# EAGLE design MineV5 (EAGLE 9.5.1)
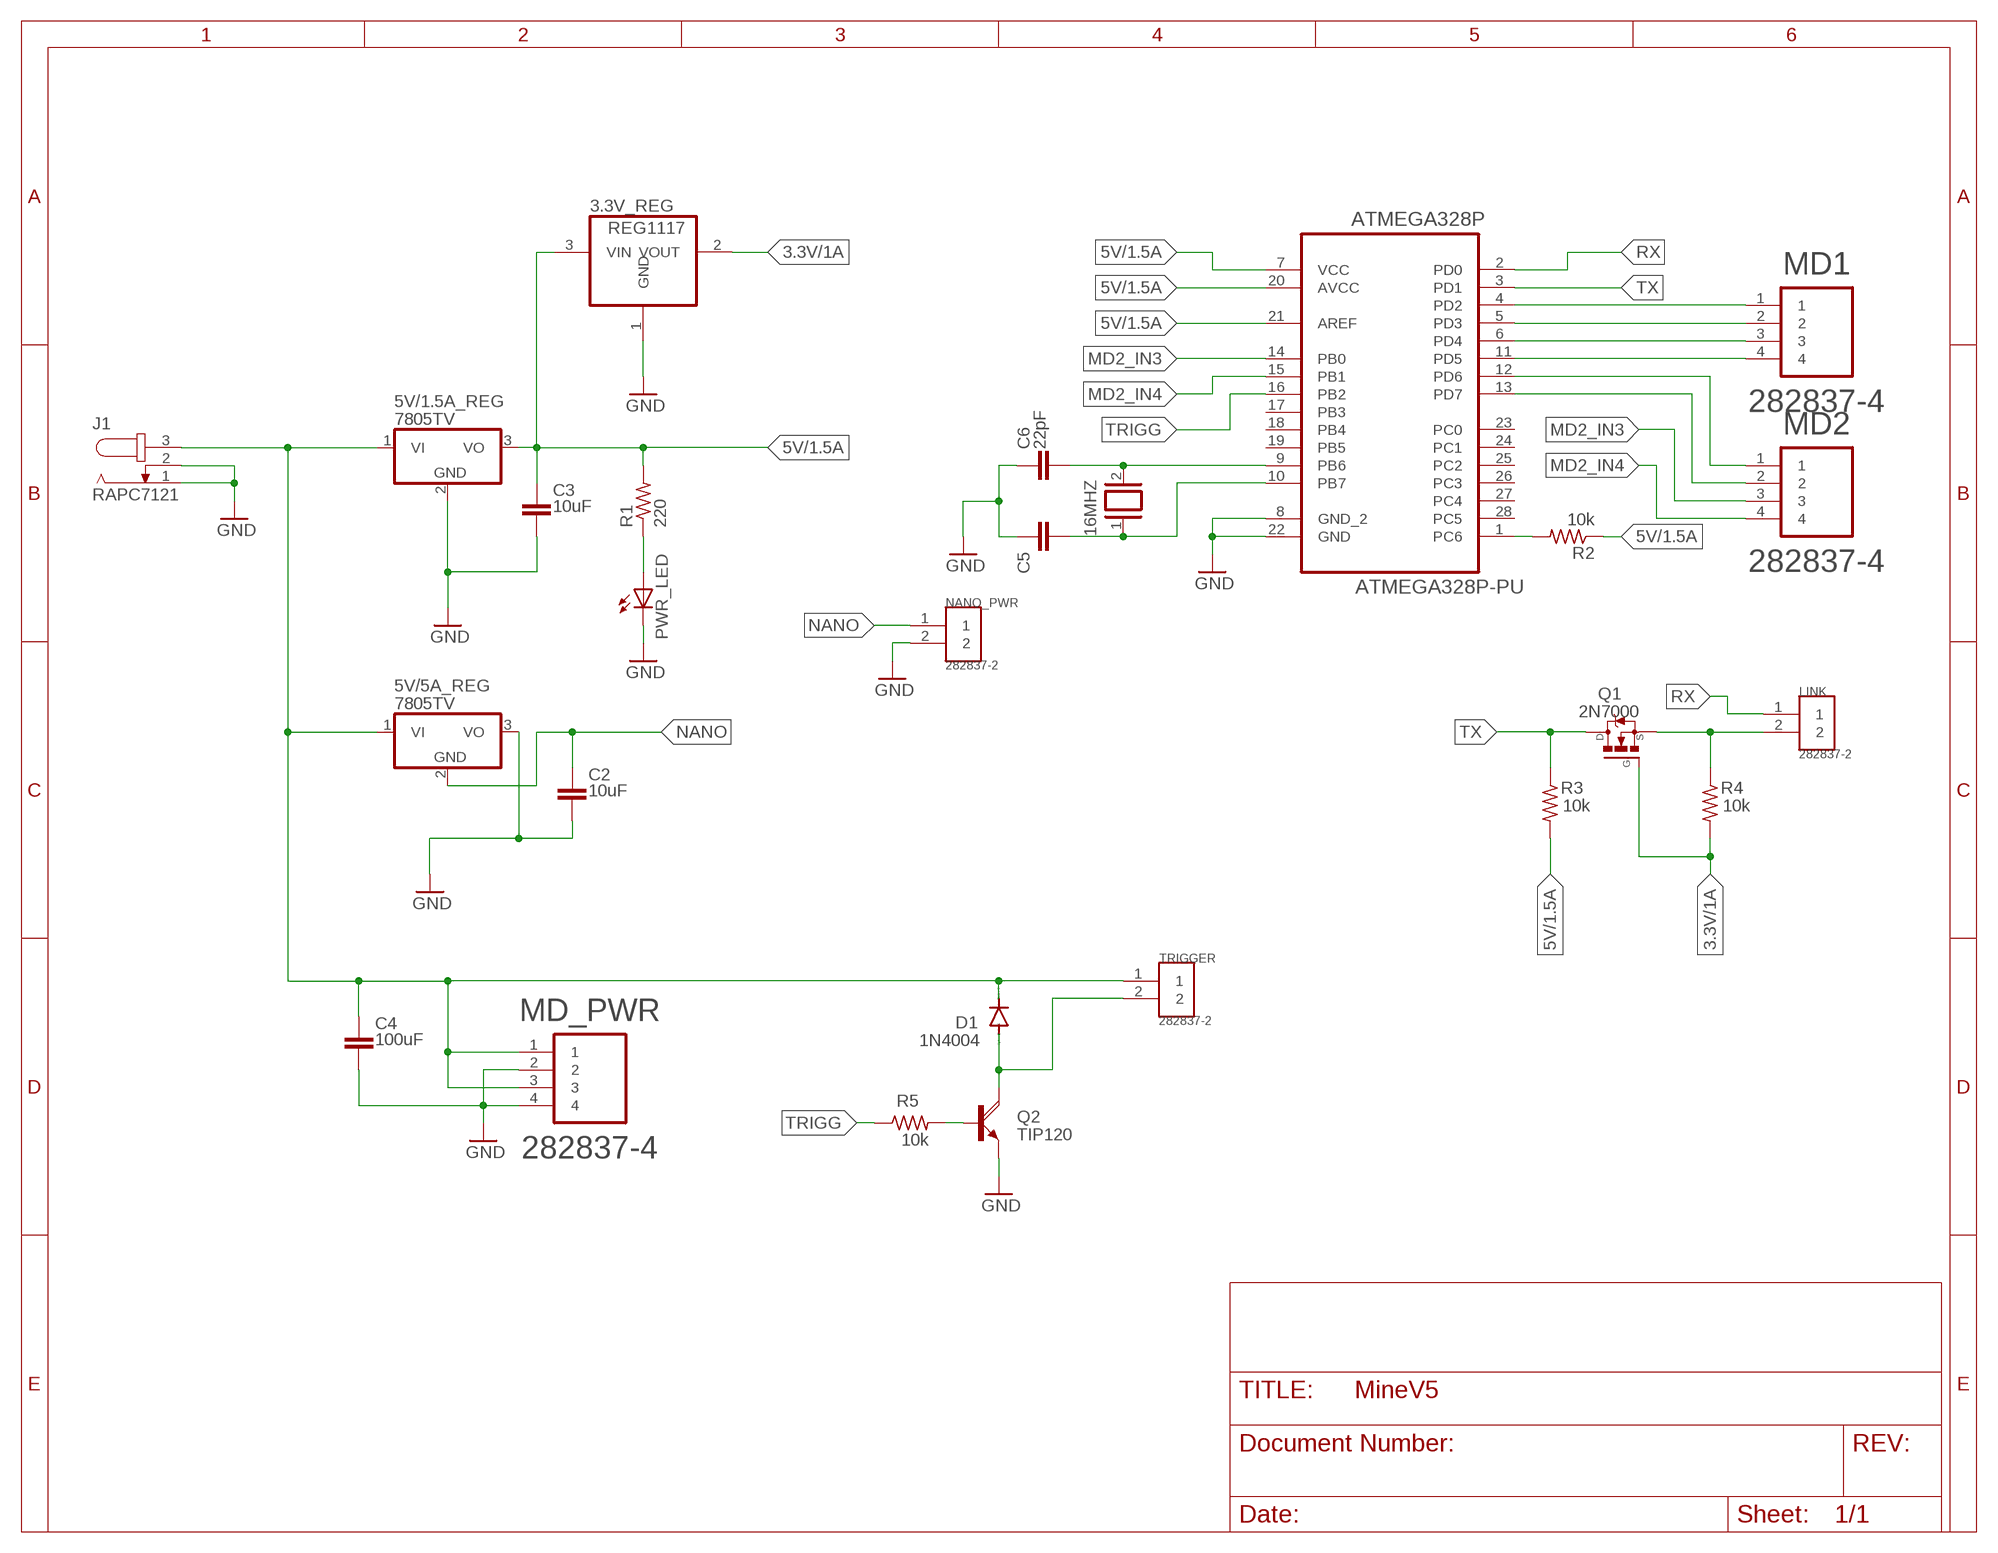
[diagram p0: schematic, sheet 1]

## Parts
3.3V_REG  REG1117  [SOT223]
5V/1.5A_REG  7805TV  [TO220V]
5V/5A_REG  7805TV  [TO220V]
16MHZ  XTAL  [Q]
ATMEGA328P  ATMEGA328P-PU  [DIP254P762X457-28]
C2  10uF  C-EU075-052X106  [C075-052X106]
C3  10uF  C-EU075-052X106  [C075-052X106]
C4  100uF  C-EU075-052X106  [C075-052X106]
C5  22pF  C-EU075-052X106  [C075-052X106]
C6  22pF  C-EU075-052X106  [C075-052X106]
D1  1N4004  [DO41-10]
J1  RAPC7121  [SPC4078]
LINK  282837-2  [TE_282837-2]
MD1  282837-4  [TE_282837-4]
MD2  282837-4  [TE_282837-4]
MD_PWR  282837-4  [TE_282837-4]
NANO_PWR  282837-2  [TE_282837-2]
PWR_LED  LEDSML1206  [SML1206]
Q1  2N7000  [TO-92]
Q2  TIP120  [TO220AH]
R1  220  R-US_R2010  [R2010]
R2  10k  R-US_R2010  [R2010]
R3  10k  R-US_R2010  [R2010]
R4  10k  R-US_R2010  [R2010]
R5  10k  R-US_R2010  [R2010]
TRIGGER  282837-2  [TE_282837-2]

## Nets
3.3V/1A: 3.3V_REG.2(VOUT) Q1.2(G) R4.2
5V/1.5A: 3.3V_REG.3(VIN) 5V/1.5A_REG.3(VO) ATMEGA328P.7(VCC) ATMEGA328P.20(AVCC) ATMEGA328P.21(AREF) C3.1 R1.2 R2.1 R3.2
GND: 3.3V_REG.1(GND) 5V/1.5A_REG.2(GND) 5V/5A_REG.3(VO) ATMEGA328P.8(GND_2) ATMEGA328P.22(GND) C2.2 C3.2 C4.2 C5.1 C6.1 J1.1 J1.2 MD_PWR.2 MD_PWR.4 NANO_PWR.2 PWR_LED.C Q2.E
MD2_IN3: ATMEGA328P.14(PB0) MD2.3
MD2_IN4: ATMEGA328P.15(PB1) MD2.4
N$1: ATMEGA328P.4(PD2) MD1.1
N$2: PWR_LED.A R1.1
N$3: 16MHZ.1 ATMEGA328P.10(PB7) C5.2
N$4: 16MHZ.2 ATMEGA328P.9(PB6) C6.2
N$5: ATMEGA328P.5(PD3) MD1.2
N$6: ATMEGA328P.6(PD4) MD1.3
N$7: ATMEGA328P.11(PD5) MD1.4
N$8: ATMEGA328P.12(PD6) MD2.1
N$9: ATMEGA328P.13(PD7) MD2.2
N$10: ATMEGA328P.1(PC6) R2.2
N$11: LINK.2 Q1.1(S) R4.1
N$12: Q2.B R5.2
N$13: 5V/1.5A_REG.1(VI) 5V/5A_REG.1(VI) C4.1 D1.C J1.3 MD_PWR.1 MD_PWR.3 TRIGGER.1
N$14: D1.A Q2.C TRIGGER.2
NANO: 5V/5A_REG.2(GND) C2.1 NANO_PWR.1
RX: ATMEGA328P.2(PD0) LINK.1
TRIGG: ATMEGA328P.16(PB2) R5.1
TX: ATMEGA328P.3(PD1) Q1.3(D) R3.1
Unconnected: ATMEGA328P.17(PB3) ATMEGA328P.18(PB4) ATMEGA328P.19(PB5) ATMEGA328P.23(PC0) ATMEGA328P.24(PC1) ATMEGA328P.25(PC2) ATMEGA328P.26(PC3) ATMEGA328P.27(PC4) ATMEGA328P.28(PC5)

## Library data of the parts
3.3V_REG = burr-brown:REG1117: 800mA and 1A Low Dropout (LDO) Positive Regulator 1.8V, 2.5V, 2.85V, 3.3V, 5V, and Adj; MPN: REG1117; OC_FARNELL: 1097566; OC_NEWARK: 14P6981
5V/1.5A_REG 5V/5A_REG = linear:78*: Positive VOLTAGE REGULATOR Source: http://cache.national.com/ds/LM/LM78L05.pdf http://www.fairchildsemi.com/ds/LM/LM7805.pdf
16MHZ = special:XTAL: CRYSTAL
ATMEGA328P = ATMEGA328P-PU:ATMEGA328P-PU: 8-bit Microcontroller with In-System Programmable Flash; AVAILABILITY: Unavailable; DESCRIPTION: Embedded microcontroller ATMEGA328P-PU PDIP 28 Microchip Technology 8-Bit 20 MHz I/O number 23; MF: Microchip; MP: ATMEGA328P-PU; PACKAGE: PDIP-28 Microchip; PRICE: None
C2-C6 = rcl:C-EU: CAPACITOR, European symbol; SPICEPREFIX: C
D1 = diode:1N4004: DIODE
J1 = RAPC712:RAPC712: DC POWER JACK Power Jack, DC, Right Angle, Through Hole, Rated 5A at 16VDC, PC Terminals Distributor: Farnell (www.Farnell.de) Drawing: 84N1161.pdf / 84N1162.pdf Manufacturer: SPC Technology (www.spctechnology.com) Type: SPC4077 / SPC 4078; AVAILABILITY: Unavailable; DESCRIPTION: Power Barrel Connector Jack 2.50mm ID _0.098_, 5.50mm OD _0.217_ Through Hole, Right Angle; MF: Switchcraft; MP: RAPC712; PACKAGE: None; PRICE: None
LINK NANO_PWR TRIGGER = 282837-2:282837-2: TERM BLOCK 5.08MM 2POS SIDE ENTY; COMMENT: 282837-2; DESCRIPTION: Connector Terminal Blocks Receptacle 2 Position 5.08mm Solder Straight Thru-Hole 13.5A/Contact; DIGI-KEY_PART_NUMBER: A113320-ND; DIGI-KEY_PURCHASE_URL: https://www.digikey.com/product-detail/en/te-connectivity-amp-connectors/282837-2/A113320-ND/2187973?utm_source=snapeda&utm_medium=aggregator&utm_campaign=symbol; MF: TE Connectivity; MP: 282837-2; PACKAGE: None; TE_PURCHASE_URL: https://www.te.com/usa-en/product-282837-2.html?te_bu=Cor&te_type=disp&te_campaign=seda_glo_cor-seda-global-disp-prtnr-fy19-seda-model-bom-cta_sma-317_1&elqCampaignId=32493
MD1 MD2 MD_PWR = 282837-4:282837-4: TERM BLOCK 5.08MM 4POS SIDE ENTY; COMMENT: 282837-4; DESCRIPTION: Conn Terminal Block F 4 POS 5.08mm Solder ST Thru-Hole 13.5A/Contact; DIGI-KEY_PART_NUMBER: A124423-ND; DIGI-KEY_PURCHASE_URL: https://www.digikey.com/product-detail/en/te-connectivity-amp-connectors/282837-4/A124423-ND/2187975?utm_source=snapeda&utm_medium=aggregator&utm_campaign=symbol; EU_ROHS_COMPLIANCE: Compliant with Exemptions; MF: TE Connectivity; MP: 282837-4; PACKAGE: None; TE_PURCHASE_URL: https://www.te.com/usa-en/product-282837-4.html?te_bu=Cor&te_type=disp&te_campaign=seda_glo_cor-seda-global-disp-prtnr-fy19-seda-model-bom-cta_sma-317_1&elqCampaignId=32493
PWR_LED = led:LED: LED
Q1 = 2N7000:2N7000: N-Channel MOSFET; AVAILABILITY: Unavailable; DESCRIPTION: N-Channel 60V 350mA _Tc_ 1W _Tc_ Through Hole TO-92-3; MF: STMicroelectronics; MP: 2N7000; PACKAGE: TO-92 ON Semiconductor; PRICE: None
Q2 = transistor-power:TIP120: NPN DARLINGTON TRANSISTOR
R1-R5 = resistor:R-US_: RESISTOR, American symbol

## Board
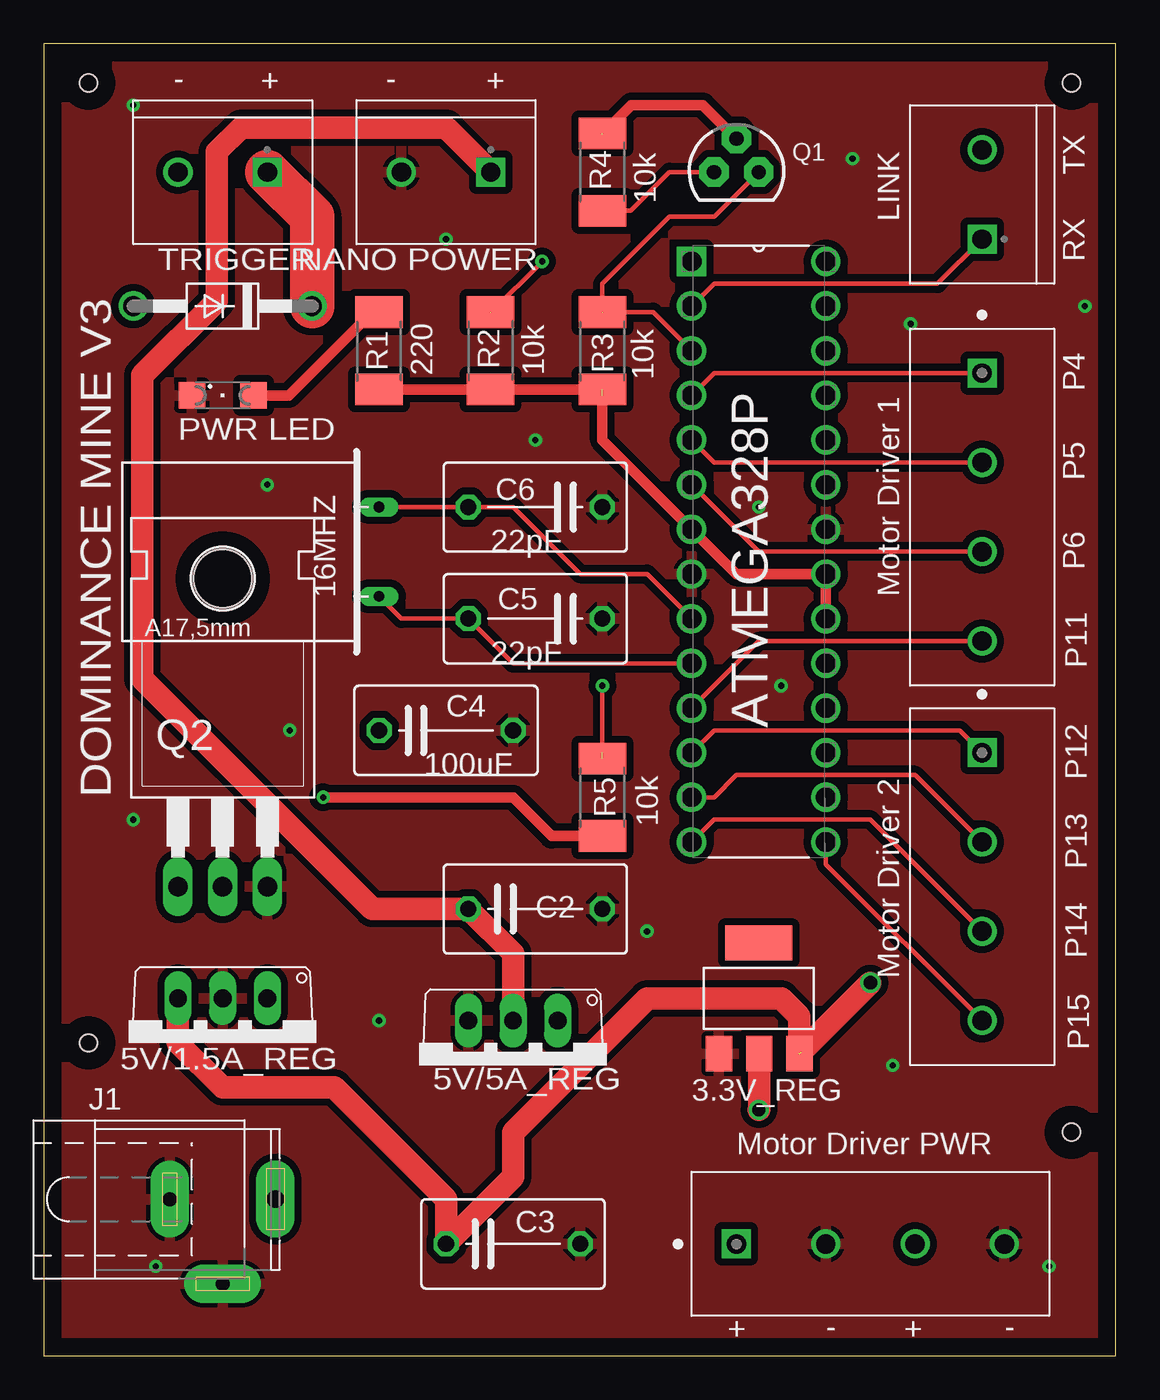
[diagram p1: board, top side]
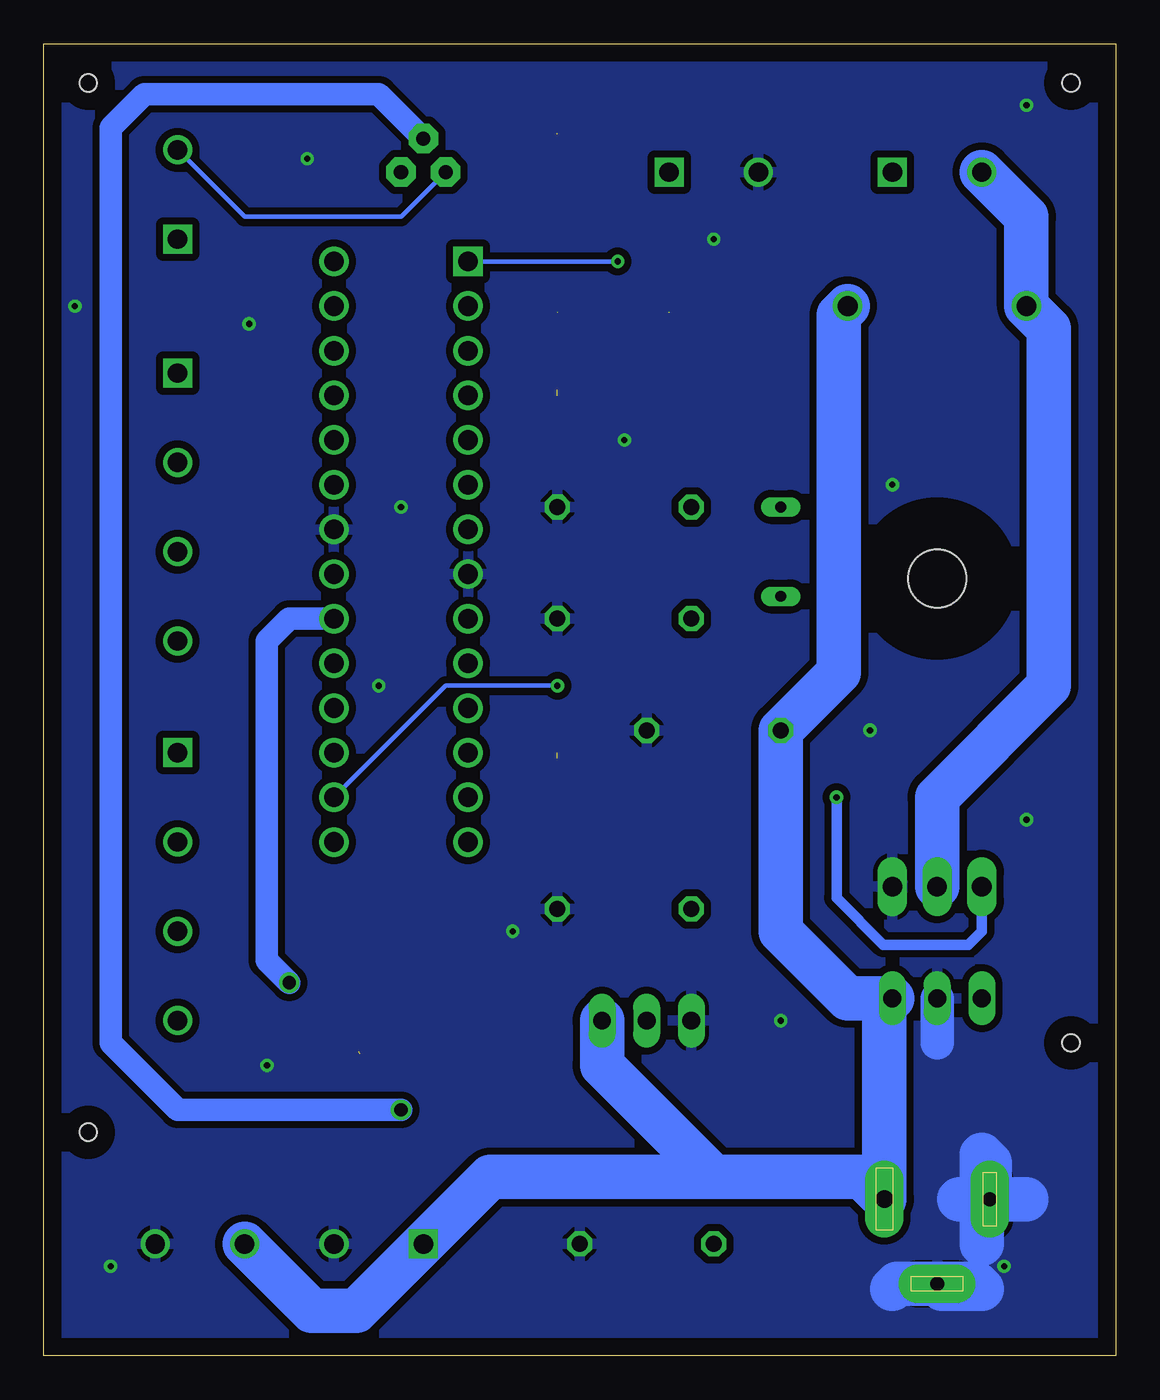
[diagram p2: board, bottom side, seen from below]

Size 60.94 x 74.6 mm. Coordinates in mm from the lower left corner, seen from the top.
Outline: 0,0 60.94,0 60.94,74.6 0,74.6 0,0
Copper layers (1*16): Top 0.035mm / dielectric 1.5mm / Bottom 0.035mm
Design rules "default": minimum track width 6mil, minimum drill 0.35mm, track to track 6mil, track to pad 6mil, pad to pad 6mil, via to via 6mil, smd to smd 6mil, copper to edge 40mil, drill to drill 6mil, minimum pad ring 10mil, minimum via ring 8mil, stop-mask expansion 4mil, vias tented up to drill 0mil, thermal gap 10mil
Holes 1 mm at 2.54,72.39 58.42,72.39 2.54,17.78 58.42,12.7

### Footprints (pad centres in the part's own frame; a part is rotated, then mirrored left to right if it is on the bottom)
SOT223 = smd 1.499 x 2.007: 1 -2.261,-3.15; 2 0.025,-3.15; 3 2.311,-3.15 | smd 3.81 x 2.007: 4 0,3.15
TO220V = drill 1.016 long: 1 -2.54,-2.54; 2 0,-2.54; 3 2.54,-2.54
Q = drill 0.61 long: 1 -2.54,-7.62; 2 2.54,-7.62
DIP254P762X457-28 = drill 1.118 square: 1 -7.62,33.02 | drill 1.118: 2 -7.62,30.48; 3 -7.62,27.94; 4 -7.62,25.4; 5 -7.62,22.86; 6 -7.62,20.32; 7 -7.62,17.78; 8 -7.62,15.24; 9 -7.62,12.7; 10 -7.62,10.16; 11 -7.62,7.62; 12 -7.62,5.08; 13 -7.62,2.54; 14 -7.62,0; 15 0,0; 16 0,2.54; 17 0,5.08; 18 0,7.62; 19 0,10.16; 20 0,12.7; 21 0,15.24; 22 0,17.78; 23 0,20.32; 24 0,22.86; 25 0,25.4; 26 0,27.94; 27 0,30.48; 28 0,33.02
C075-052X106 = drill 0.914 octagon: 1 -3.81,0; 2 3.81,0
DO41-10 = drill 1.118: A 5.08,0; C -5.08,0
SPC4078 = drill 0.8 pad 2.184 long: 1 -3,0; 2 0,-4.8 | drill 1 pad 2.184 long: 3 3,0
TE_282837-2 = drill 1.1 square: 1 -2.54,0 | drill 1.1: 2 2.54,0
TE_282837-4 = drill 1.1 square: 1 0,0 | drill 1.1: 2 5.08,0; 3 10.16,0; 4 15.24,0
SML1206 = smd 1.5 x 1.5: A 1.75,0; C -1.75,0
TO-92 = drill 0.813 pad 1.676 octagon: 1 -1.27,0; 2 0,1.905; 3 1.27,0
TO220AH = drill 1.118 long: B -2.54,-6.35; C 0,-6.35; E 2.54,-6.35 | hole 3.302: 0,11.176
R2010 = smd 1.8 x 2.7: 1 -2.2,0; 2 2.2,0

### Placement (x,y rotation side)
3.3V_REG  40.64,20.32 0 top
5V/1.5A_REG  10.16,17.78 180 top
5V/5A_REG  26.67,16.51 180 top
16MHZ  11.43,45.72 90 top
ATMEGA328P  44.45,29.21 0 top
C2  27.94,25.4 0 top
C3  26.67,6.35 0 top
C4  22.86,35.56 0 top
C5  27.94,41.91 180 top
C6  27.94,48.26 180 top
D1  10.16,59.69 180 top
J1  10.16,8.89 0 top
LINK  53.34,66.04 90 top
MD1  53.34,55.88 270 top
MD2  53.34,34.29 270 top
MD_PWR  39.37,6.35 0 top
NANO_PWR  22.86,67.31 180 top
PWR_LED  10.16,54.61 0 top
Q1  39.37,67.31 0 top
Q2  10.16,33.02 0 top
R1  19.05,57.15 270 top
R2  25.4,57.15 90 top
R3  31.75,57.15 270 top
R4  31.75,67.31 90 top
R5  31.75,31.75 270 top
TRIGGER  10.16,67.31 180 top

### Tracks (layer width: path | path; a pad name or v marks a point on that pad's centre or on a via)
3.3V/1A  (via drill 0.75)  (1 unrouted)
  Top 0.61: Q1.2 37.47,71.12 33.4,71.12 31.75,69.47
  Top 1.27: 40.64,17.2 3.3V_REG.2 40.66,13.99 v40.64,13.97
  Bottom 1.27: Q1.2 41.91,71.75 55.24,71.75 57.15,69.85 57.15,17.78 53.34,13.97 v40.64,13.97
5V/1.5A  (via drill 0.75)  (2 unrouted)
  Top 0.61: R1.2 R2.1 R3.2 | 31.75,54.61 31.75,52.07 ATMEGA328P.7 39.37,44.45 ATMEGA328P.21 ATMEGA328P.20
  Top 1.27: 5V/1.5A_REG.3 7.62,17.78 10.16,15.24 16.51,15.24 22.86,8.89 C3.1 26.67,10.16 26.67,12.7 34.29,20.32 41.91,20.32 42.95,19.28 3.3V_REG.3 | v46.99,21.21 43.05,17.27
  Bottom 1.27: ATMEGA328P.20 46.99,41.91 48.26,40.64 48.26,22.48 v46.99,21.21
GND  (via drill 0.35)
  Bottom 1.905: 5V/1.5A_REG.2 10.16,17.78
  Bottom 2.54: J1.1 8.89,8.89 | J1.1 7.16,10.97 7.62,11.43 7.62,9.35 J1.1 | J1.1 7.62,8.43 7.62,6.35 | J1.1 5.08,8.89 | J1.2 7.9,4.09 7.62,3.81 9.88,3.81 J1.2 | J1.2 12.42,4.09 12.7,3.81
  other vias: 13.97,35.56 12.7,49.53 27.94,52.07 22.86,63.5 5.08,71.12 45.97,68.07 49.28,58.67 48.26,16.51 57.15,5.08 34.29,24.13 19.05,19.05 6.35,5.08 40.64,48.26 5.08,30.48 41.91,38.1 59.18,59.69
  pour Top (isolate 0.406): 0,74.93 60.96,74.93 60.96,0 0,0
  pour Bottom (isolate 0.406): 0,74.93 60.96,74.93 60.96,0 0,0
MD2_IN3
  Top 0.254: MD2.3 46.99,30.48 38.1,30.48 ATMEGA328P.14
MD2_IN4
  Top 0.254: MD2.4 44.45,27.94 ATMEGA328P.15
N$1
  Top 0.254: ATMEGA328P.4 38.1,55.88 MD1.1
N$2
  Top 0.61: R1.1 18.67,59.35 15.2,55.88 13.93,54.61 PWR_LED.A
N$3
  Top 0.254: ATMEGA328P.10 26.67,39.37 C5.2 20.32,41.91 16MHZ.1
N$4
  Top 0.254: 16MHZ.2 C6.2 26.67,48.26 30.48,44.45 34.29,44.45 ATMEGA328P.9
N$5
  Top 0.254: ATMEGA328P.5 38.1,50.8 MD1.2
N$6
  Top 0.254: MD1.3 40.64,45.72 ATMEGA328P.6
N$7
  Top 0.254: MD1.4 40.64,40.64 ATMEGA328P.11
N$8
  Top 0.254: MD2.1 52.07,35.56 38.1,35.56 ATMEGA328P.12
N$9
  Top 0.254: MD2.2 49.53,33.02 39.37,33.02 38.1,31.75 ATMEGA328P.13
N$10  (via drill 0.35)  (1 unrouted)
  Top 0.254: v28.32,62.23 25.4,59.31
  Bottom 0.254: ATMEGA328P.1 v28.32,62.23
N$11
  Top 0.254: R4.1 33.36,65.11 35.56,67.31 Q1.1
  Bottom 0.254: Q1.1 40.64,64.77 49.53,64.77 LINK.2
N$12  (via drill 0.35)
  Top 0.61: R5.2 28.87,29.55 26.67,31.75 v15.88,31.75
  Bottom 0.61: Q2.B 7.62,24.13 8.38,23.37 13.21,23.37 15.88,26.04 v15.88,31.75
N$13
  Top 2.54: TRIGGER.1 15.24,64.77 D1.C
  Bottom 2.54: D1.C 15.75,59.18 15.75,38.86 C4.1 19.05,24.13 15.24,20.32 5V/1.5A_REG.1 13.16,19.86 J1.3 14.43,10.16 22.86,10.16 | 5V/5A_REG.1 29.21,16.51 22.86,10.16 | MD_PWR.3 45.72,2.54 43.18,2.54 MD_PWR.1 35.56,10.16 22.86,10.16
N$14
  Bottom 2.54: TRIGGER.2 5.08,64.77 D1.A 3.81,58.42 3.81,38.1 10.16,31.75 Q2.C
NANO
  Top 1.27: NANO_PWR.1 22.86,69.85 11.21,69.85 9.82,68.46 9.82,59.98 5.59,55.75 5.59,38.48 18.67,25.4 C2.1 26.67,22.86 5V/5A_REG.2
RX
  Top 0.254: LINK.1 50.8,60.96 38.1,60.96 ATMEGA328P.2
TRIGG  (via drill 0.35)  (1 unrouted)
  Top 0.254: v31.75,38.1 31.75,34.29
  Bottom 0.254: ATMEGA328P.16 38.1,38.1 v31.75,38.1
TX  (1 unrouted)
  Top 0.254: Q1.3 38.1,64.77 35.56,64.77 31.75,60.96 31.75,59.31 | R3.1 34.63,59.35 ATMEGA328P.3

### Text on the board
tPlace: - | + | - | + | TX | RX | P4 | P5 | P6 | P11 | P12 | P13 | P14 | P15 | + | - | + | -
tNames: 10k | LINK | NANO POWER | TRIGGER | 220 | 10k | 10k | PWR LED | 22pF | Motor Driver 1 | 22pF | 100uF | DOMINANCE MINE V3 | 10k | Motor Driver 2 | 5V/1.5A_REG | 5V/5A_REG | Motor Driver PWR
